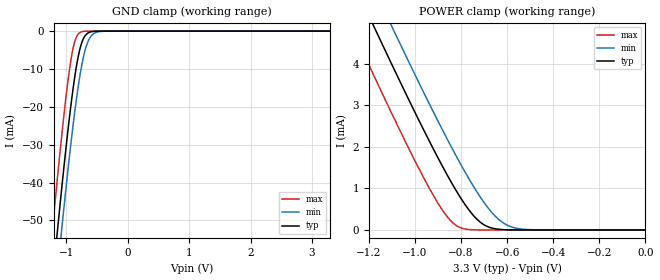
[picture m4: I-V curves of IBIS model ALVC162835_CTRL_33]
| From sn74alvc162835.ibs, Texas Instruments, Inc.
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[Model]   ALVC162835_CTRL_33
Model_type  Input
Vinl=0.8
Vinh=2.0
| variable   typ   min   max
C_comp   11.60pF   11.12pF   11.85pF
[Temperature Range]   40   100   -40
| Ambient temperature   25   85   -40
[Voltage range]   3.3   3   3.6
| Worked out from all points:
|   GND clamp passes 1 mA (typ) near -0.68 V on its own axis
|   POWER clamp passes 1 mA (typ) near -0.83 V on its own axis
[GND Clamp]
| ALVC162835_CTRL_33
|   Voltage   I(typ)   I(min)   I(max)
-3.3V     -451.4mA   -460.2mA   -440.6mA
-1.225V   -66.77mA   -77.63mA   -52.81mA
-1.14V    -52.55mA   -63.42mA   -38.55mA
-1.07V    -41.27mA   -52.08mA   -27.39mA
-975mV    -26.91mA   -37.4mA    -13.81mA
-905mV    -17.45mA   -27.36mA   -6.068mA
-845mV    -10.58mA   -19.54mA   -2.069mA
-765mV    -4.1mA     -10.78mA   -298.6uA
-700mV    -1.444mA   -5.604mA   -52.39uA
-640mV    -472.1uA   -2.617mA   -10.24uA
-470mV    -15.62uA   -178.3uA   -98.79nA
3.3V      1.114nA    76.54nA    5.893pA
[POWER Clamp]
| ALVC162835_CTRL_33
|   Voltage   I(typ)   I(min)   I(max)
-3.3V     31.15mA    32.01mA    30.07mA
-1.275V   6.052mA    6.966mA    4.871mA
-1.185V   4.979mA    5.895mA    3.795mA
-1.145V   4.507mA    5.423mA    3.323mA
-1.105V   4.038mA    4.953mA    2.855mA
-1.07V    3.632mA    4.545mA    2.451mA
-940mV    2.164mA    3.062mA    1.029mA
-845mV    1.174mA    2.029mA    223.2uA
-730mV    253.2uA    906.9uA    1.947uA
-630mV    13.46uA    223.6uA    15.19nA
-520mV    261.9nA    13.16uA    81.04pA
-48.03fV  1.114nA    59.61nA    6.941pA
